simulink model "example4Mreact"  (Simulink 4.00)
settings: Solver=ode45  StartTime=0.0  StopTime=20.0  RelTol=1e-3

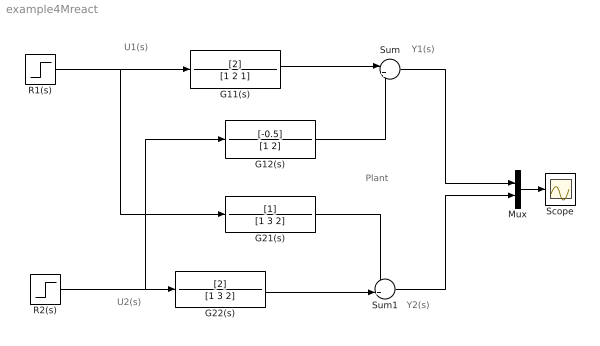
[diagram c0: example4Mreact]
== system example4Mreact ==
  note: Y1(s)
  note: Y2(s)
  note: U1(s)
  note: U2(s)
  note: Plant
  G11(s) : TransferFcn  Numerator=[2]  Denominator=[1 2 1]  AbsoluteTolerance=auto  Realization=auto
  G12(s) : TransferFcn  Numerator=[-0.5]  Denominator=[1 2]  AbsoluteTolerance=auto  Realization=auto
  G21(s) : TransferFcn  Numerator=[1]  Denominator=[1 3 2]  AbsoluteTolerance=auto  Realization=auto
  G22(s) : TransferFcn  Numerator=[2]  Denominator=[1 3 2]  AbsoluteTolerance=auto  Realization=auto
  Mux : Mux  Inputs=2
  R1(s) : Step  Time=1  Before=0  After=1  SampleTime=0
  R2(s) : Step  Time=5  Before=0  After=-1  SampleTime=0
  Scope : Scope
  Sum : Sum  Inputs=|++  SaturateOnIntegerOverflow=on
  Sum1 : Sum  Inputs=++|  SaturateOnIntegerOverflow=on
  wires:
  G11(s)/1 -> Sum/1
  Sum/1 -> Mux/1
  G22(s)/1 -> Sum1/2
  Sum1/1 -> Mux/2
  G12(s)/1 -> Sum/2
  G21(s)/1 -> Sum1/1
  R1(s)/1 -> G11(s)/1, G21(s)/1
  R2(s)/1 -> G22(s)/1, G12(s)/1
  Mux/1 -> Scope/1
